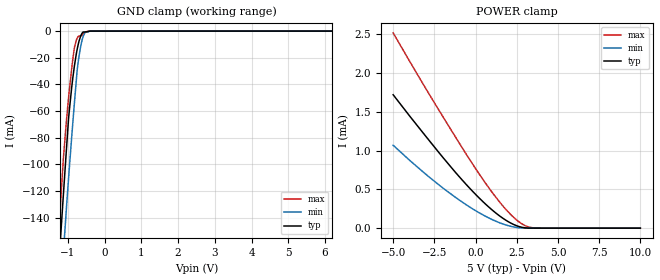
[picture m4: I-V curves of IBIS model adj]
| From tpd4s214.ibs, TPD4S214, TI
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|   adj Model
[Model]   adj
Model_type   Input
Vinl = 0.4
Vinh = 1.2
|   typ   min   max
|   (nom PVT)   (fast PVT)   (slow PVT)
C_comp   1.404e-12   1.365e-12   1.458e-12
| Where nom  PVT is Nominal Process, 5V, 27C
|   Fast PVT is Strong Process,  5.5V, -40C
|   Slow PVT is Weak Process,   4.5V, 125C
[Voltage Range]   5   4.5   5.5
|Junction Temperature
[Temperature Range]   27   125   -40
[Power Clamp Reference]   5   4.5   5.5
[GND Clamp Reference]   0   0   0
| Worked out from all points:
|   GND clamp passes 1 mA (typ) near -0.59 V on its own axis
[GND Clamp]
|   Voltage   I(typ)   I(min)   I(max)
-5V       -1.949A    -1.93A     -1.973A
-1.252V   -177.8mA   -220.6mA   -153.2mA
-1.121V   -123.1mA   -166.6mA   -95.87mA
-1.046V   -92.21mA   -136.1mA   -70.1mA
-980mV    -66mA      -110.8mA   -50.37mA
-895mV    -42.54mA   -79.85mA   -28.33mA
-820mV    -26.12mA   -53.95mA   -12.3mA
-743mV    -13.42mA   -28.8mA    -5.188mA
-715mV    -9.845mA   -22.82mA   -4.043mA
-581mV    -679.3uA   -3.888mA   -2.116mA
-400mV    -7.444uA   0A         0A
10V       0A         0A         0A
[POWER Clamp]
|   Voltage   I(typ)   I(min)   I(max)
-5V       1.721mA    1.069mA    2.519mA
-3.911V   1.423mA    858.7uA    2.12mA
-2.294V   993.8uA    570.2uA    1.546mA
-1.25V    727.6uA    402.2uA    1.187mA
-182mV    476.2uA    249.6uA    828.1uA
670mV     297.9uA    146.2uA    560.7uA
1.369V    172.4uA    77.34uA    361.5uA
2.092V    70.8uA     26.26uA    184.8uA
2.591V    23.96uA    6.432uA    88.67uA
3.035V    3.731uA    581nA      29.79uA
3.445V    498.3nA    174.3nA    5.749uA
10V       0A         0A         0A
